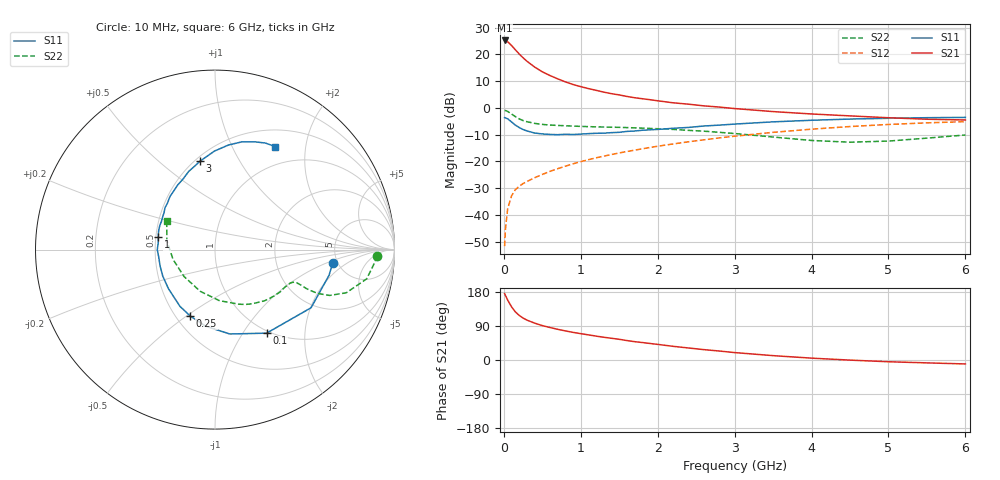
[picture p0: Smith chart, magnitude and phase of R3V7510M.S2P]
! SIEMENS Small Signal Semiconductors
! BFR181
! Si NPN RF Bipolar Junction Transistor in SOT23
! VCE = 0.75 V  IC = 10 mA
! Common Emitter S-Parameters:  May  1996
# GHz  S  MA  R  50
!  f  S11  S21  S12  S22
! GHz  MAG  ANG  MAG  ANG  MAG  ANG  MAG  ANG
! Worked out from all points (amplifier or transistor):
!   36 points, 10 MHz to 6 GHz, reference 50 ohm
!   highest |S21| = 25.2 dB at 10 MHz (marker M1)
!   |S21| within 3 dB of that: start of sweep to 134.7 MHz
!   unconditionally stable (mu >= 1): start of sweep to 11.82 MHz; 312.3 MHz to end of sweep
!   at 250 MHz: K = 0.89, MSG = 23.5 dB, |S12| = -28.3 dB
!   at 1.4 GHz: K = 1.41, MAG = 7.6 dB, |S12| = -17.4 dB
!   at 6 GHz: K = 1.11, MAG = -1.7 dB, |S12| = -5.1 dB
!   S11 on the Smith chart (normalised r, x): 10 MHz: 4.52, -1.23; 100 MHz: 0.97, -1.29; 250 MHz: 0.59, -0.52; 1 GHz: 0.52, +0.08; 3 GHz: 0.53, +0.69; 6 GHz: 0.73, +1.49
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0.01  0.6592 -6.7  18.27 175.5  0.0026 82.8  0.9026 -2.2
0.02  0.6516 -12.6  18.05 170.8  0.0053 84.5  0.8928 -4.6
0.05  0.6257 -31.2  17.27 158.0  0.0131 75.4  0.8609 -10.9
0.1  0.5472 -58.3  14.72 140.4  0.0227 65.8  0.77 -18.2
0.15  0.4773 -80.1  12.21 126.9  0.0296 59.9  0.6878 -21.8
0.2  0.4298 -97.0  10.21 117.7  0.0343 57.8  0.6239 -23.1
0.25  0.3949 -110.4  8.657 110.7  0.0385 57.1  0.5803 -23.2
0.3  0.3718 -121.6  7.478 105.3  0.0421 58.1  0.553 -23.1
0.4  0.3391 -139.6  5.822 97.3  0.0495 59.3  0.5147 -22.4
0.5  0.3266 -152.9  4.736 90.8  0.057 61.4  0.4914 -22.1
0.6  0.3194 -163.2  4.032 85.7  0.0652 62.4  0.4786 -22.3
0.7  0.3162 -172.1  3.498 81.0  0.0731 64.0  0.4707 -22.8
0.8  0.3216 -180.0  3.07 76.8  0.0813 64.3  0.464 -23.4
1  0.324 167.4  2.5 69.5  0.0989 65.7  0.4518 -25.5
1.1  0.3308 161.7  2.3 66.3  0.1077 65.9  0.4471 -26.8
1.6  0.3637 139.9  1.639 51.3  0.1531 64.7  0.429 -34.3
2.2  0.416 119.9  1.247 36.1  0.212 61.1  0.3969 -45.9
3  0.4988 99.8  0.973 19.6  0.2958 53.3  0.3323 -66.3
3.5  0.5491 90.3  0.854 11.5  0.3496 47.3  0.2855 -85.1
4.5  0.6192 75.9  0.71 -0.3  0.4488 33.5  0.2285 -139.0
5.5  0.6567 64.7  0.615 -7.6  0.526 19.2  0.2725 169.7
6  0.665 59.6  0.595 -10.4  0.5542 11.7  0.3119 149.6
